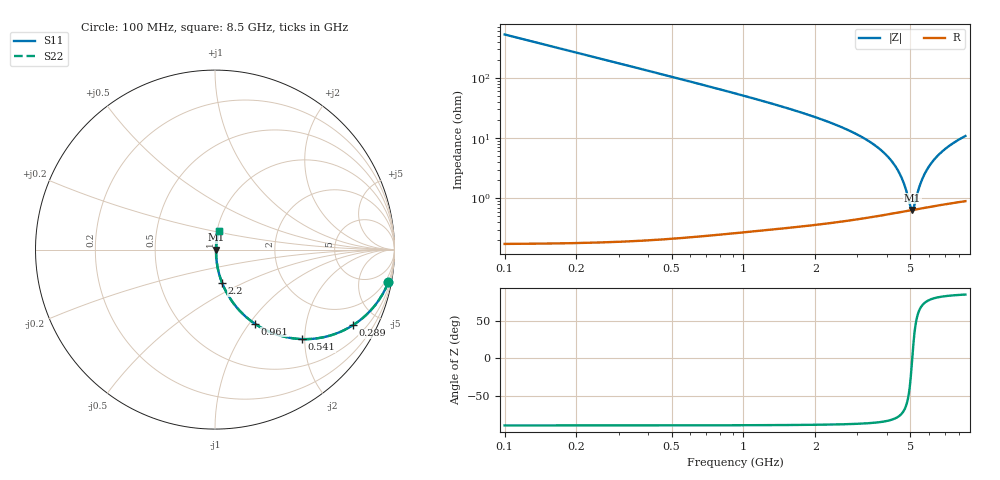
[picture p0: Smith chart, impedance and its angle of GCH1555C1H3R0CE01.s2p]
!Murata Part Number: GCH1555C1H3R0CE01
!These Parameters are Measured in Series Mode Connection
!Data Generated on Mar 13, 2026
!  o--ll--o
!Port1  Port2
!  o------o
!Operation Temp=25[degC], DC Bias Voltage=0[V]
!Freq. Start=100[MHz] Stop=9[GHz] 401[Steps]
# Hz S RI R 50
!Freq.(Hz) S11(Real) S11(Imag) S21(Real) S21(Imag) S12(Real) S12(Imag) S22(Real) S22(Imag)
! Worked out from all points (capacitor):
!   401 points, 100 MHz to 8.5 GHz, reference 50 ohm
!   read as one part in series: C = 3 pF near 142 MHz
!   lowest |Z| = 638 mohm at 5.098 GHz (marker M1)
!   series resonance near 5.093 GHz, so ESL is about 330 pH
!   S11 on the Smith chart (normalised r, x): 100 MHz: 1, -11; 289 MHz: 1.00, -3.66; 541 MHz: 1.00, -1.94; 961 MHz: 1.01, -1.06; 2.2 GHz: 1.01, -0.39; 8.5 GHz: 1.02, +0.22
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1e8  0.9656 -0.1821  0.0344 0.1821  0.0344 0.1821  0.9656 -0.1821
2.05e8  0.8695 -0.3365  0.1305 0.3365  0.1305 0.3365  0.8695 -0.3365
2.89e8  0.7697 -0.4205  0.2303 0.4205  0.2303 0.4205  0.7697 -0.4205
4.15e8  0.6168 -0.4854  0.3832 0.4854  0.3832 0.4854  0.6168 -0.4854
5.41e8  0.4841 -0.4986  0.5159 0.4986  0.5159 0.4986  0.4841 -0.4986
7.3e8  0.3362 -0.4707  0.6638 0.4707  0.6638 0.4707  0.3362 -0.4707
9.61e8  0.2213 -0.4126  0.7787 0.4126  0.7787 0.4126  0.2213 -0.4126
1.507e9  0.0953 -0.2887  0.9047 0.2887  0.9047 0.2887  0.0953 -0.2887
2.2e9  0.04 -0.1865  0.96 0.1865  0.96 0.1865  0.04 -0.1865
2.914e9  0.0187 -0.1187  0.9813 0.1187  0.9813 0.1187  0.0187 -0.1187
3.733e9  0.00924 -0.0641  0.9908 0.0641  0.9908 0.0641  0.00924 -0.0641
4.3e9  0.00681 -0.0345  0.9932 0.0345  0.9932 0.0345  0.00681 -0.0345
4.636e9  0.00629 -0.0191  0.9937 0.0191  0.9937 0.0191  0.00629 -0.0191
4.783e9  0.00622 -0.0127  0.9938 0.0127  0.9938 0.0127  0.00622 -0.0127
5.014e9  0.00627 -0.00316  0.9937 0.00316  0.9937 0.00316  0.00627 -0.00316
5.098e9  0.00633 0.000201  0.9937 -0.000201  0.9937 -0.000201  0.00633 0.000201
5.182e9  0.00642 0.0035  0.9936 -0.0035  0.9936 -0.0035  0.00642 0.0035
5.455e9  0.00684 0.0139  0.9932 -0.0139  0.9932 -0.0139  0.00684 0.0139
5.707e9  0.00739 0.023  0.9926 -0.023  0.9926 -0.023  0.00739 0.023
6.274e9  0.00911 0.0421  0.9909 -0.0421  0.9909 -0.0421  0.00911 0.0421
7.114e9  0.0126 0.0678  0.9874 -0.0678  0.9874 -0.0678  0.0126 0.0678
8.5e9  0.0201 0.1052  0.9799 -0.1052  0.9799 -0.1052  0.0201 0.1052
